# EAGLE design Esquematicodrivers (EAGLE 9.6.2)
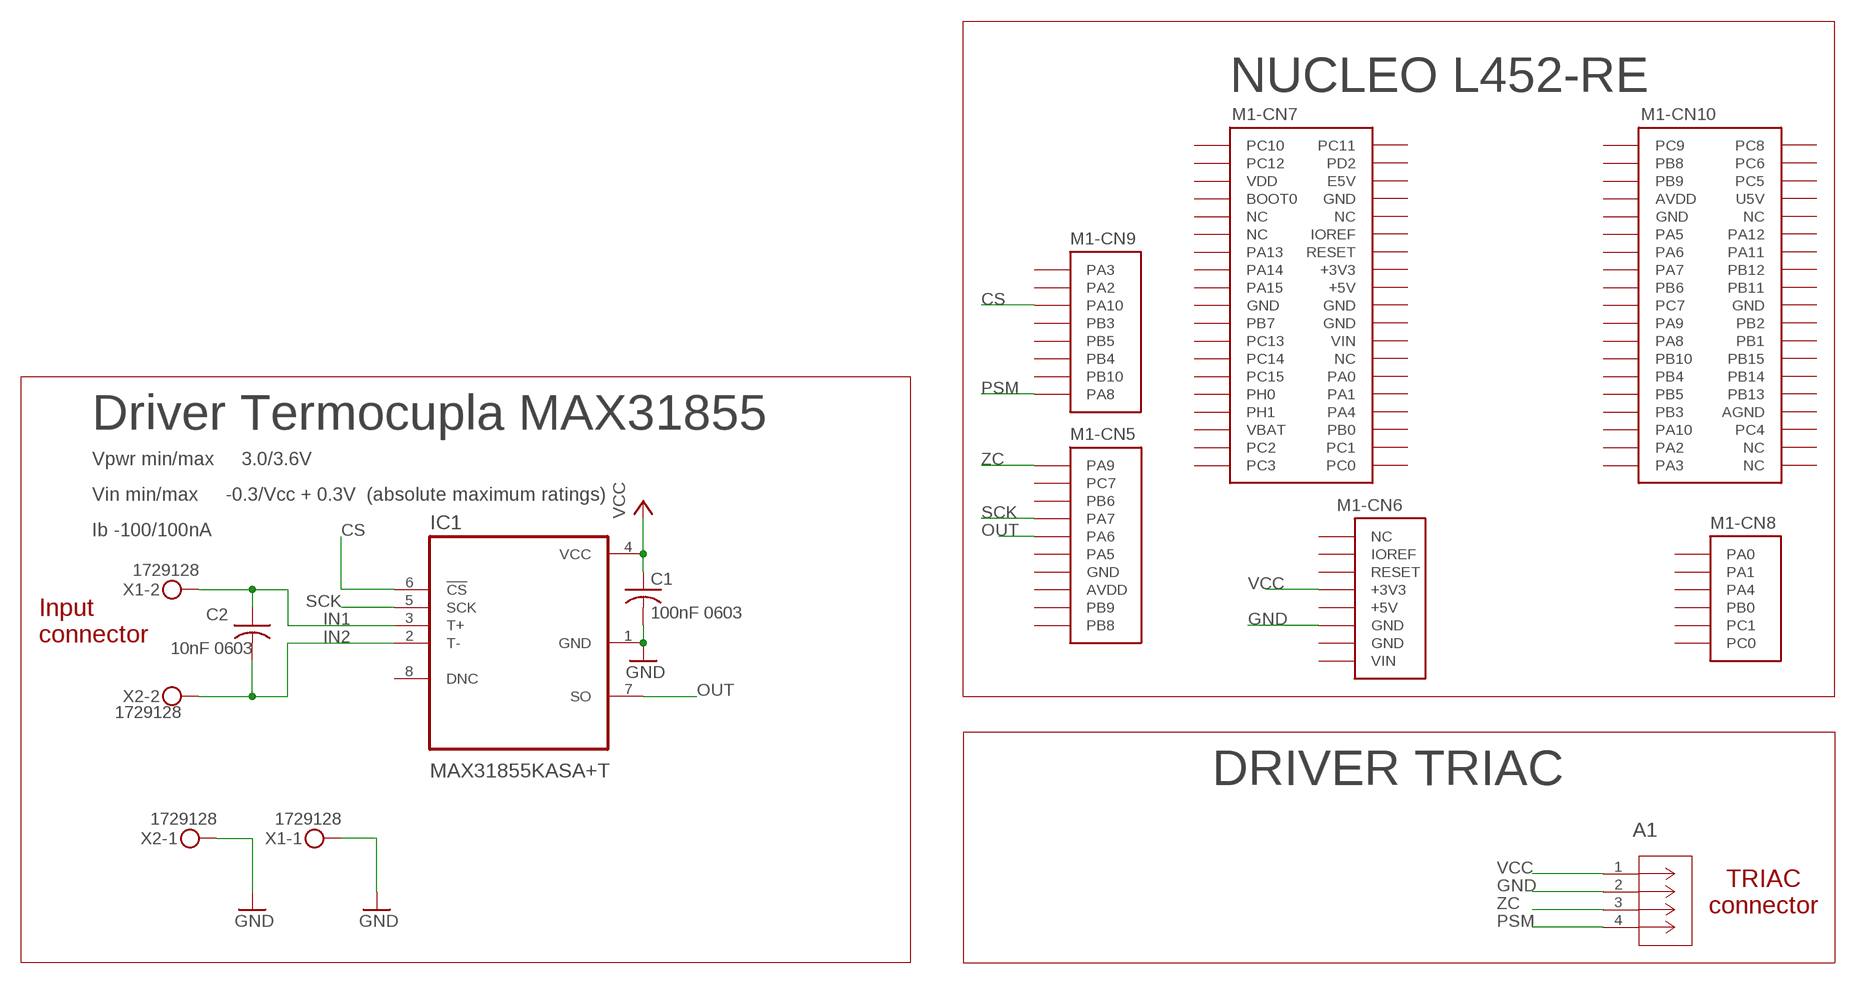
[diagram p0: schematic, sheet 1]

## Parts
A1  PPTC041LFBN-RC  PPTC041LFBN-RCCONN_PPTC041LFBN-RC_SUL  [CONN_PPTC041LFBN-RC_SUL]
C1  100nF 0603  C-USC0603  [C0603]
C2  10nF 0603  C-USC0603  [C0603]
IC1  MAX31855KASA+T  [SOIC127P600X175-8N]
M1  HDR-ETD  NUCLEO-L452RE  [NUCLEO-64]
X1  1729128  MKDSN1,5/2-5,08  [MKDSN1,5/2-5,08]
X2  1729128  MKDSN1,5/2-5,08  [MKDSN1,5/2-5,08]

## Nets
CS: IC1.6(!CS) M1.CN9-3(-CN9:PA10)
GND: A1.2(GND) C1.2 IC1.1(GND) M1.CN6-6(-CN6:GND) X1.1 X2.1
IN1: C2.1 IC1.3(T+) X1.2
IN2: C2.2 IC1.2(T-) X2.2
OUT: IC1.7(SO) M1.CN5-5(-CN5:PA6)
PSM: A1.4(PWM) M1.CN9-8(-CN9:PA8)
SCK: IC1.5(SCK) M1.CN5-4(-CN5:PA7)
VCC: A1.1(VCC) C1.1 IC1.4(VCC) M1.CN6-4(-CN6:+3V3)
ZC: A1.3(Z-C) M1.CN5-1(-CN5:PA9)
Unconnected: IC1.8(DNC) M1.CN5-2(-CN5:PC7) M1.CN5-3(-CN5:PB6) M1.CN5-6(-CN5:PA5) M1.CN5-9(-CN5:PB9) M1.CN5-10(-CN5:PB8) M1.CN6-1(-CN6:NC) M1.CN6-3(-CN6:RESET) M1.CN7-1(-CN7:PC10) M1.CN7-2(-CN7:PC11) M1.CN7-3(-CN7:PC12) M1.CN7-4(-CN7:PD2) M1.CN7-6(-CN7:E5V) M1.CN7-7(-CN7:BOOT0) M1.CN7-9(-CN7:NC) M1.CN7-10(-CN7:NC) M1.CN7-11(-CN7:NC) M1.CN7-12(-CN7:IOREF) M1.CN7-13(-CN7:PA13) M1.CN7-14(-CN7:RESET) M1.CN7-15(-CN7:PA14) M1.CN7-17(-CN7:PA15) M1.CN7-21(-CN7:PB7) M1.CN7-23(-CN7:PC13) M1.CN7-25(-CN7:PC14) M1.CN7-26(-CN7:NC) M1.CN7-27(-CN7:PC15) M1.CN7-28(-CN7:PA0) M1.CN7-29(-CN7:PH0) M1.CN7-30(-CN7:PA1) M1.CN7-31(-CN7:PH1) M1.CN7-32(-CN7:PA4) M1.CN7-34(-CN7:PB0) M1.CN7-35(-CN7:PC2) M1.CN7-36(-CN7:PC1) M1.CN7-37(-CN7:PC3) M1.CN7-38(-CN7:PC0) M1.CN8-1(-CN8:PA0) M1.CN8-2(-CN8:PA1) M1.CN8-3(-CN8:PA4) M1.CN8-4(-CN8:PB0) M1.CN8-5(-CN8:PC1) M1.CN8-6(-CN8:PC0) M1.CN9-1(-CN9:PA3) M1.CN9-2(-CN9:PA2) M1.CN9-4(-CN9:PB3) M1.CN9-5(-CN9:PB5) M1.CN9-6(-CN9:PB4) M1.CN9-7(-CN9:PB10) M1.CN10-1(-CN10:PC9) M1.CN10-2(-CN10:PC8) M1.CN10-3(-CN10:PB8) M1.CN10-4(-CN10:PC6) M1.CN10-5(-CN10:PB9) M1.CN10-6(-CN10:PC5) M1.CN10-10(-CN10:NC) M1.CN10-11(-CN10:PA5) M1.CN10-12(-CN10:PA12) M1.CN10-13(-CN10:PA6) M1.CN10-14(-CN10:PA11) M1.CN10-15(-CN10:PA7) M1.CN10-16(-CN10:PB12) M1.CN10-17(-CN10:PB6) M1.CN10-18(-CN10:PB11) M1.CN10-19(-CN10:PC7) M1.CN10-21(-CN10:PA9) M1.CN10-22(-CN10:PB2) M1.CN10-23(-CN10:PA8) M1.CN10-24(-CN10:PB1) M1.CN10-25(-CN10:PB10) M1.CN10-26(-CN10:PB15) M1.CN10-27(-CN10:PB4) M1.CN10-28(-CN10:PB14) M1.CN10-29(-CN10:PB5) M1.CN10-30(-CN10:PB13) M1.CN10-31(-CN10:PB3) M1.CN10-33(-CN10:PA10) M1.CN10-34(-CN10:PC4) M1.CN10-35(-CN10:PA2) M1.CN10-36(-CN10:NC) M1.CN10-37(-CN10:PA3) M1.CN10-38(-CN10:NC)

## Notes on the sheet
- NUCLEO L452-RE
- Driver Termocupla MAX31855
- Vpwr min/max     3.0/3.6V
- Vin min/max     -0.3/Vcc + 0.3V  (absolute maximum ratings)
- Ib -100/100nA
- Input
  connector
- DRIVER TRIAC
- TRIAC
  connector

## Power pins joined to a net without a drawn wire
+3V3: M1.CN7-16(-CN7:+3V3)
+5V: M1.CN6-5(-CN6:+5V) M1.CN7-18(-CN7:+5V)
AGND: M1.CN10-32(-CN10:AGND)
AVDD: M1.CN5-8(-CN5:AVDD) M1.CN10-7(-CN10:AVDD)
GND: M1.CN5-7(-CN5:GND) M1.CN6-7(-CN6:GND) M1.CN7-8(-CN7:GND) M1.CN7-19(-CN7:GND) M1.CN7-20(-CN7:GND) M1.CN7-22(-CN7:GND) M1.CN10-9(-CN10:GND) M1.CN10-20(-CN10:GND)
IOREF: M1.CN6-2(-CN6:IOREF)
U5V: M1.CN10-8(-CN10:U5V)
VBAT: M1.CN7-33(-CN7:VBAT)
VDD: M1.CN7-5(-CN7:VDD)
VIN: M1.CN6-8(-CN6:VIN) M1.CN7-24(-CN7:VIN)

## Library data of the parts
A1 = PPTC041LFBN-RC:PPTC041LFBN-RC; COPYRIGHT: Copyright (C) 2023 Ultra Librarian. All rights reserved.; MANUFACTURER_PART_NUMBER: PPTC041LFBN-RC; MFR_NAME: Sullins; PARTNO: PPTC041LFBN-RC
C1 = rcl:C-US: CAPACITOR, American symbol; PARTNO: CC0603KRX7R7BB104; SPICEPREFIX: C
C2 = rcl:C-US: CAPACITOR, American symbol; PARTNO: GRM033R71A103KA01D; SPICEPREFIX: C
IC1 = MAX31855KASA+T-DK:MAX31855KASA+T; PARTNO: MAX31855KASA+T
M1 = NUCLEO-L452RE:NUCLEO-L452RE: No existe un outline (Layer Dimension) para esta librería. En su lugar se utilizó una referencia en tDocu. Al momento de diseñar la tarjeta, el Dimension debe ser dibujado según los requerimientos del usuario, o simplemente copiar los contenidos del tDocu en Dimensions.; PARTNO: HDR-ETD
X1 X2 = 1729128-PHOENIX CONTACT:MKDSN1,5/2-5,08: MKDSN 1,5/ 2-5,08 Printklemme; PARTNO: 1729128

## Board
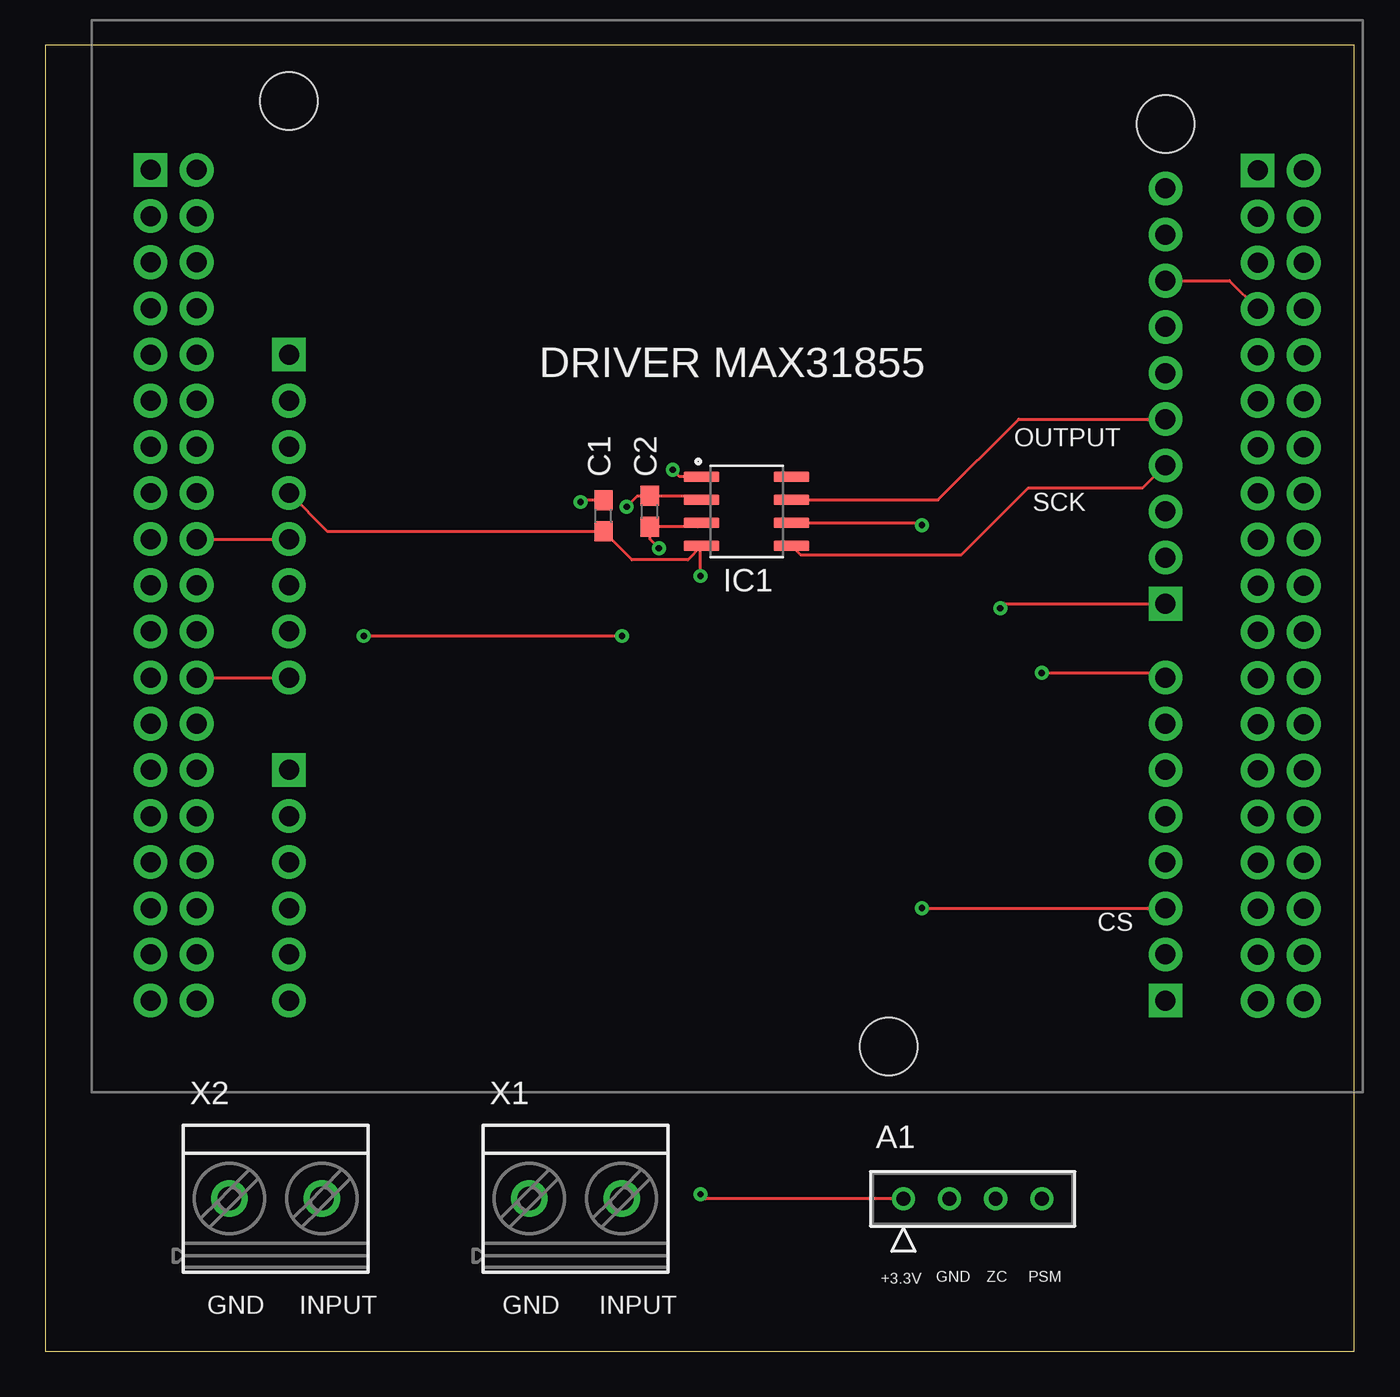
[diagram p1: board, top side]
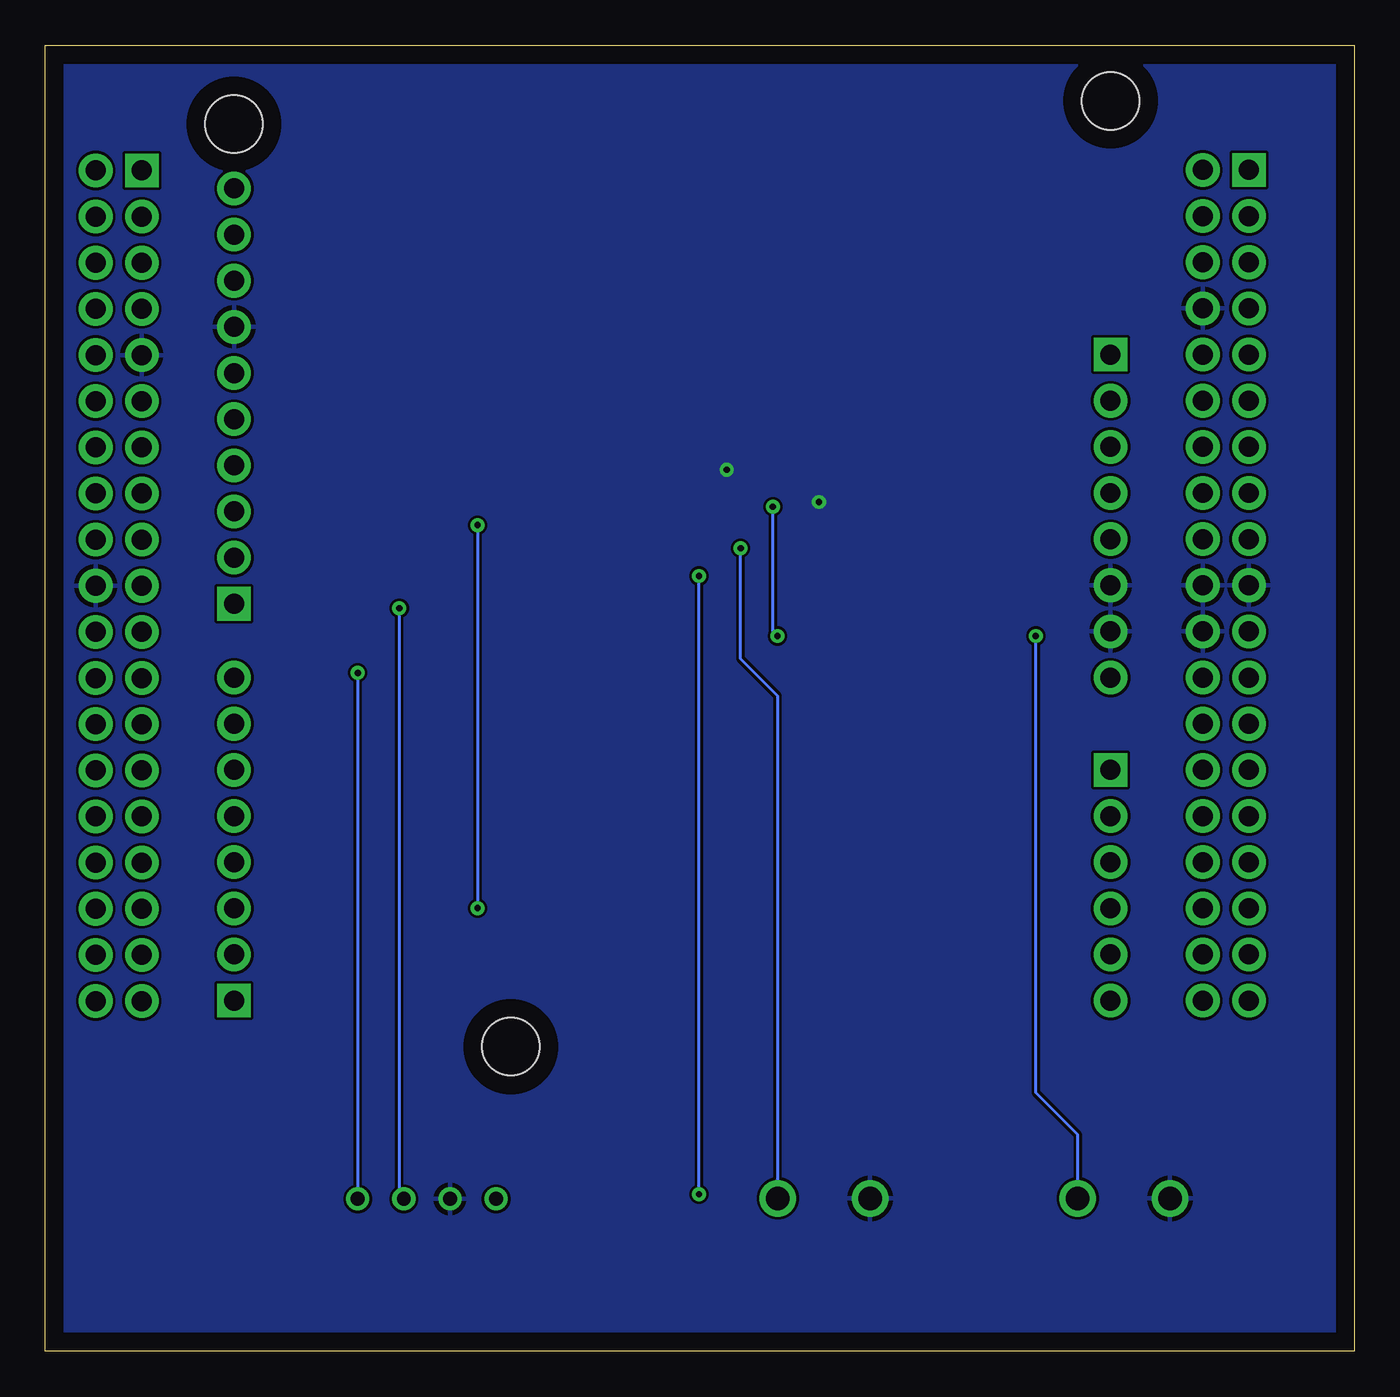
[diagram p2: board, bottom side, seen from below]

Size 72.06 x 71.87 mm. Coordinates in mm from the lower left corner, seen from the top.
Outline: 0,0 72.06,0 72.06,71.87 0,71.87 0,0
Copper layers (1*16): Top 0.035mm / dielectric 1.5mm / Bottom 0.035mm
Design rules "default *": minimum track width 6mil, minimum drill 0.3mm, track to track 6mil, track to pad 6mil, pad to pad 6mil, via to via 6mil, smd to smd 6mil, copper to edge 40mil, drill to drill 6mil, minimum pad ring 10mil, minimum via ring 8mil, stop-mask expansion 2mil, vias tented up to drill 15mil, thermal gap 10mil

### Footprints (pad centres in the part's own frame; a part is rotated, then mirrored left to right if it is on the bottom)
CONN_PPTC041LFBN-RC_SUL = drill 0.762 pad 1.27: 1 0,0; 2 -2.54,0; 3 -5.08,0; 4 -7.62,0
C0603 = smd 1.1 x 1: 1 -0.85,0; 2 0.85,0
SOIC127P600X175-8N = smd 1.97 x 0.59: 1 -2.475,1.905; 2 -2.475,0.635; 3 -2.475,-0.635; 4 -2.475,-1.905; 5 2.475,-1.905; 6 2.475,-0.635; 7 2.475,0.635; 8 2.475,1.905
NUCLEO-64 = drill 1.1 pad 1.85 square: CN5-1 59.13,24.884; CN6-1 10.87,38.6; CN7-1 3.25,48.76; CN8-1 10.87,15.74; CN9-1 59.13,3.04; CN10-1 64.21,48.735 | drill 1.1 pad 1.85: CN5-2 59.13,27.424; CN5-3 59.13,29.964; CN5-4 59.13,32.504; CN5-5 59.13,35.044; CN5-6 59.13,37.584; CN5-7 59.13,40.124; CN5-8 59.13,42.664; CN5-9 59.13,45.204; CN5-10 59.13,47.744; CN6-2 10.87,36.06; CN6-3 10.87,33.52; CN6-4 10.87,30.98; CN6-5 10.87,28.44; CN6-6 10.87,25.9; CN6-7 10.87,23.36; CN6-8 10.87,20.82; CN7-2 5.79,48.76; CN7-3 3.25,46.22; CN7-4 5.79,46.22; CN7-5 3.25,43.68; CN7-6 5.79,43.68; CN7-7 3.25,41.14; CN7-8 5.79,41.14; CN7-9 3.25,38.6; CN7-10 5.79,38.6; CN7-11 3.25,36.06; CN7-12 5.79,36.06; CN7-13 3.25,33.52; CN7-14 5.79,33.52; CN7-15 3.25,30.98; CN7-16 5.79,30.98; CN7-17 3.25,28.44; CN7-18 5.79,28.44; CN7-19 3.25,25.9; CN7-20 5.79,25.9; CN7-21 3.25,23.36; CN7-22 5.79,23.36; CN7-23 3.25,20.82; CN7-24 5.79,20.82; CN7-25 3.25,18.28; CN7-26 5.79,18.28; CN7-27 3.25,15.74; CN7-28 5.79,15.74; CN7-29 3.25,13.2; CN7-30 5.79,13.2; CN7-31 3.25,10.66; CN7-32 5.79,10.66; CN7-33 3.25,8.12; CN7-34 5.79,8.12; CN7-35 3.25,5.58; CN7-36 5.79,5.58; CN7-37 3.25,3.04; CN7-38 5.79,3.04; CN8-2 10.87,13.2; CN8-3 10.87,10.66; CN8-4 10.87,8.12; CN8-5 10.87,5.58; CN8-6 10.87,3.04; CN9-2 59.13,5.58; CN9-3 59.13,8.12; CN9-4 59.13,10.66; CN9-5 59.13,13.2; CN9-6 59.13,15.74; CN9-7 59.13,18.28; CN9-8 59.13,20.82; CN10-2 66.75,48.735; CN10-3 64.21,46.195; CN10-4 66.75,46.195; CN10-5 64.21,43.655; CN10-6 66.75,43.655; CN10-7 64.21,41.115; CN10-8 66.75,41.115; CN10-9 64.21,38.575; CN10-10 66.75,38.575; CN10-11 64.21,36.035; CN10-12 66.75,36.035; CN10-13 64.21,33.495; CN10-14 66.75,33.495; CN10-15 64.21,30.955; CN10-16 66.75,30.955; CN10-17 64.21,28.415; CN10-18 66.75,28.415; CN10-19 64.21,25.875; CN10-20 66.75,25.875; CN10-21 64.21,23.335; CN10-22 66.75,23.335; CN10-23 64.21,20.795; CN10-24 66.75,20.795; CN10-25 64.21,18.255; CN10-26 66.75,18.255; CN10-27 64.21,15.715; CN10-28 66.75,15.715; CN10-29 64.21,13.175; CN10-30 66.75,13.175; CN10-31 64.21,10.635; CN10-32 66.75,10.635; CN10-33 64.21,8.095; CN10-34 66.75,8.095; CN10-35 64.21,5.555; CN10-36 66.75,5.555; CN10-37 64.21,3.015; CN10-38 66.75,3.015 | hole 3.175: 59.13,51.3; 10.87,52.57; 43.89,0.5
MKDSN1,5/2-5,08 = drill 1.3 pad 2: 1 -2.561,0.025; 2 2.519,0.025

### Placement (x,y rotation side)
A1  47.24,8.38 180 top
C1  30.73,45.97 90 top
C2  33.27,46.23 90 top
IC1  38.61,46.23 0 top
M1  2.54,16.26 0 top
X1  29.21,8.38 0 top
X2  12.7,8.38 0 top

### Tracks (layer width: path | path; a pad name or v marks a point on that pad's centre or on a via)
+5V
  Top 0.152: M1.CN7-18 M1.CN6-5
AVDD
  Top 0.152: M1.CN5-8 65.2,58.92 M1.CN10-7
CS  (via drill 0.35)
  Top 0.152: IC1.6 48.13,45.59 v48.26,45.47 | v48.26,24.38 61.66,24.38 M1.CN9-3
  Bottom 0.152: v48.26,45.47 v48.26,24.38
GND  (via drill 0.35)
  Top 0.152: IC1.1 34.93,48.13 v34.54,48.51 | C1.2 29.55,46.82 v29.46,46.74
  pour Bottom: 0,71.88 72.39,71.88 72.39,-0.25 0,-0.25
  pour Bottom: 1.52,71.88 71.88,71.88 71.88,0 1.52,0
IN1  (via drill 0.35)
  Top 0.152: IC1.3 35.92,45.38 C2.1 33.27,44.7 v33.78,44.2
  Bottom 0.152: v33.78,44.2 33.78,38.1 31.75,36.07 31.75,8.43 X1.2
IN2  (via drill 0.35)
  Top 0.152: v32,46.48 32.6,47.08 C2.2 35.47,47.08 35.81,46.74 | v17.53,39.37 v31.75,39.37
  Top 0.254: 35.81,46.74 36.01,46.74 IC1.2
  Bottom 0.152: v31.75,39.37 32,39.62 v32,46.48 | X2.2 15.22,11.92 17.53,14.22 v17.53,39.37
OUT
  Top 0.152: IC1.7 49.15,46.86 53.59,51.31 M1.CN5-5
PSM  (via drill 0.35)
  Top 0.152: v54.86,37.34 61.41,37.34 M1.CN9-8
  Bottom 0.152: v54.86,37.34 A1.4
SCK
  Top 0.152: IC1.5 41.59,43.81 50.42,43.81 54.1,47.5 60.41,47.5 M1.CN5-4
VCC  (via drill 0.35)
  Top 0.152: M1.CN6-4 15.52,45.12 C1.1 32.3,43.56 35.37,43.56 IC1.4 36.07,44.26 v36.07,42.67 | A1.1 36.32,8.38 v36.07,8.64
  Bottom 0.152: v36.07,8.64 v36.07,42.67
VIN
  Top 0.152: M1.CN7-24 M1.CN6-8
ZC  (via drill 0.35)
  Top 0.152: v52.58,40.89 52.82,41.14 M1.CN5-1
  Bottom 0.152: A1.3 52.58,8.64 v52.58,40.89

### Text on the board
tPlace: DRIVER MAX31855 | OUTPUT | SCK | CS | +3.3V | GND | ZC | PSM | GND | INPUT | GND | INPUT
tNames: A1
